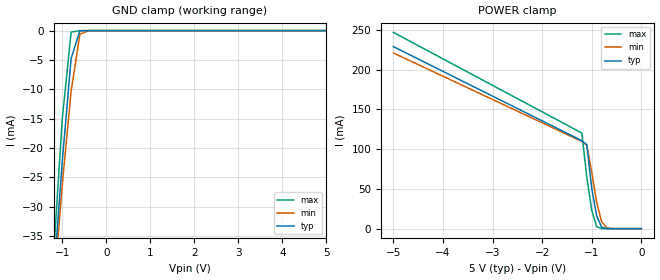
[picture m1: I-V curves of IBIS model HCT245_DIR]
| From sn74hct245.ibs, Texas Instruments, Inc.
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|   Model HCT245_DIR
[Model]   HCT245_DIR
Model_type  Input
Polarity   Inverting
Vinl = 0.8
Vinh = 2.0
| variable   typ   min   max
C_comp   3.0pf   NA   10pf
[Temperature Range]   25   85   -40
[Voltage Range]   5.0   4.5   5.5
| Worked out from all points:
|   GND clamp passes 1 mA (typ) near -0.64 V on its own axis
|   POWER clamp passes 1 mA (typ) near -0.75 V on its own axis
[GND Clamp]
|   Voltage   I(typ)   I(min)   I(max)
-5V       -550.7mA   -500.3mA   -603.1mA
-1.2V     -42.47mA   -44.69mA   -38.42mA
-1V       -22.21mA   -26.22mA   -14.96mA
-800mV    -4.751mA   -10.32mA   -247uA
-600mV    -20.76uA   -612.2uA   -2.366uA
-400mV    -10.84nA   -3.135uA   -2.152uA
5V        53.54pA    6.747uA    2.613uA
[POWER Clamp]
|   Voltage   I(typ)   I(min)   I(max)
-5V       229mA      221mA      246.9mA
-1.2V     110.7mA    109.8mA    120.3mA
-1.1V     105.6mA    104.8mA    64.63mA
-1V       50.32mA    70.94mA    22.88mA
-900mV    15.78mA    32.55mA    2.352mA
-800mV    1.871mA    8.77mA     47.82uA
-700mV    101.9uA    1.173mA    4.034uA
-600mV    3.153uA    106.6uA    3.575uA
0V        335.4pA    195.2nA    304.7nA
